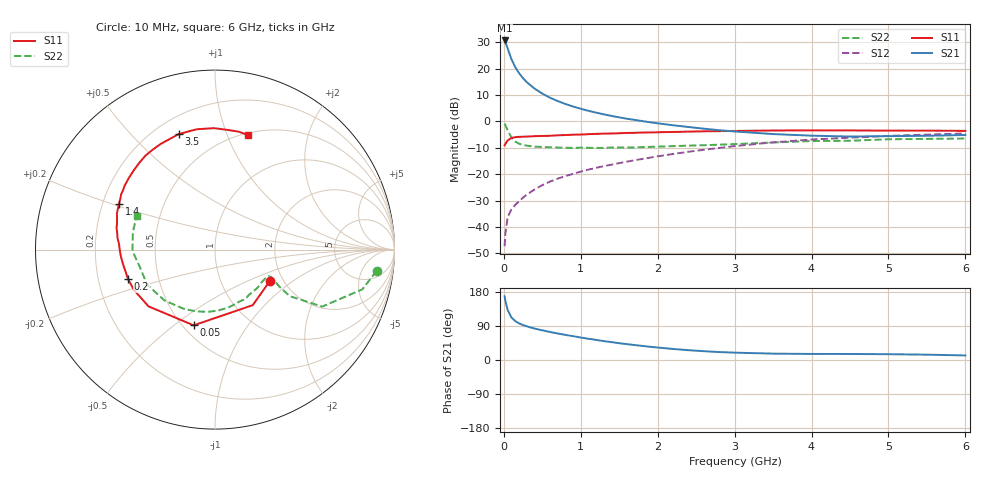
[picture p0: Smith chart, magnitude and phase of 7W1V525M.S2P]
! Infineon Technologies  Discrete & RF Semiconductors
! BFS17W
! Si NPN RF Bipolar Junction Transistor in SOT323
! VCE = 1.5 V  IC = 25 mA
! Common Emitter S-Parameters:  August  1999
# GHz  S  MA  R  50
!  f  S11  S21  S12  S22
! GHz  MAG  ANG  MAG  ANG  MAG  ANG  MAG  ANG
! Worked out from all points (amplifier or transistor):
!   36 points, 10 MHz to 6 GHz, reference 50 ohm
!   highest |S21| = 30.8 dB at 10 MHz (marker M1)
!   |S21| within 3 dB of that: start of sweep to 48.9 MHz
!   unconditionally stable (mu >= 1): 138.2 MHz to end of sweep
!   at 250 MHz: K = 1.29, MAG = 19.4 dB, |S12| = -28.9 dB
!   at 1.4 GHz: K = 1.42, MAG = 5.4 dB, |S12| = -16.4 dB
!   at 6 GHz: K = 1.13, MAG = -2.4 dB, |S12| = -4.6 dB
!   S11 on the Smith chart (normalised r, x): 10 MHz: 1.70, -0.69; 50 MHz: 0.57, -0.59; 200 MHz: 0.33, -0.15; 1.4 GHz: 0.27, +0.21; 3.5 GHz: 0.29, +0.69; 6 GHz: 0.52, +1.19
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0.01  0.352 -30.2  34.53 168.0  0.0043 77.3  0.908 -7.5
0.02  0.3742 -55.8  32.5 156.3  0.0075 70.8  0.8503 -15.1
0.05  0.4383 -105.7  24.18 131.6  0.0154 59.7  0.6764 -28.0
0.1  0.4871 -139.5  15.08 112.0  0.0216 54.9  0.491 -31.9
0.15  0.5045 -153.5  10.63 102.4  0.0262 55.7  0.4134 -29.9
0.2  0.5114 -161.1  8.182 96.5  0.0309 60.7  0.379 -27.9
0.25  0.5135 -166.7  6.611 92.2  0.036 61.2  0.3585 -26.5
0.3  0.5181 -170.3  5.549 88.7  0.0412 64.1  0.348 -26.1
0.4  0.5262 -176.1  4.205 82.9  0.0514 66.3  0.3333 -26.3
0.5  0.5314 179.7  3.381 78.3  0.0619 68.0  0.3282 -27.5
0.6  0.536 176.5  2.827 74.0  0.0723 69.0  0.3231 -29.5
0.7  0.5466 173.4  2.444 70.0  0.0823 69.3  0.3202 -32.2
0.9  0.5614 167.6  1.923 62.9  0.1016 69.7  0.3157 -38.3
1.1  0.5744 161.8  1.593 56.0  0.1221 69.7  0.3165 -45.2
1.4  0.592 154.5  1.278 47.2  0.1517 69.4  0.3201 -56.6
1.8  0.6168 144.8  1.018 37.1  0.1945 68.3  0.3263 -72.5
2.2  0.6328 135.5  0.848 29.1  0.2418 66.1  0.3408 -87.7
2.8  0.6559 122.0  0.683 21.0  0.3151 60.7  0.3627 -110.4
3.5  0.6746 107.5  0.577 16.8  0.402 52.5  0.3996 -134.9
4.5  0.6767 90.5  0.518 15.9  0.492 39.0  0.4305 -167.4
5.5  0.6701 78.6  0.536 14.1  0.5627 27.6  0.468 167.9
6  0.6646 73.9  0.554 12.0  0.5917 22.1  0.4748 156.9
